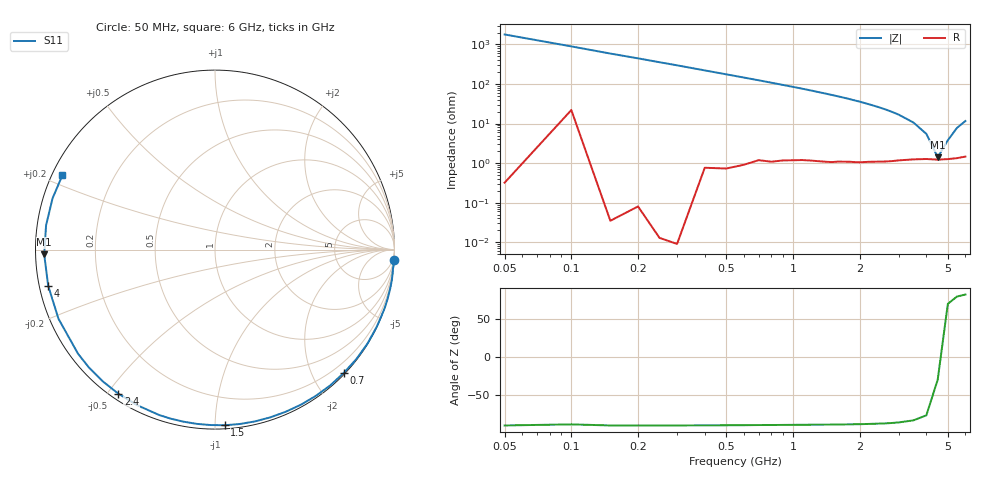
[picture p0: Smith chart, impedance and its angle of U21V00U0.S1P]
! SIEMENS Discrete & RF Semiconductors
! BBY52-02W
! Si Tuning Diode in SCD-80
! VR = 1 V
! S-Parameters:  September  1997
# GHz  S  MA  R  50
!  f  S11
! GHz  MAG  ANG
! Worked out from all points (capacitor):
!   34 points, 50 MHz to 6 GHz, reference 50 ohm
!   read as one part to ground: C = 1.78 pF near 50 MHz
!   lowest |Z| = 1.41 ohm at 4.5 GHz (marker M1)
!   series resonance near 4.582 GHz, so ESL is about 680 pH
!   S11 on the Smith chart (normalised r, x): 50 MHz: 0, -36; 700 MHz: 0.02, -2.49; 1.5 GHz: 0.02, -1.06; 2.4 GHz: 0.02, -0.53; 4 GHz: 0.03, -0.11; 6 GHz: 0.03, +0.23
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0.05  1 -3.2
0.2  1 -12.8
0.3  1 -19.1
0.4  0.9985 -25.5
0.5  0.9978 -31.7
0.6  0.9962 -37.8
0.7  0.9934 -43.8
0.8  0.9923 -49.7
0.9  0.9899 -55.5
1  0.9879 -61.0
1.1  0.9857 -66.4
1.2  0.9841 -71.8
1.3  0.9828 -77.0
1.5  0.9801 -86.8
1.6  0.9778 -91.5
1.8  0.9747 -100.4
2  0.9726 -108.7
2.2  0.9692 -116.6
2.4  0.9666 -123.8
2.6  0.9643 -130.5
2.8  0.9617 -136.9
3  0.9586 -142.8
3.5  0.9534 -156.2
4  0.9509 -167.8
4.5  0.9521 -178.4
5  0.9509 171.8
5.5  0.949 162.5
6  0.9458 154.0
